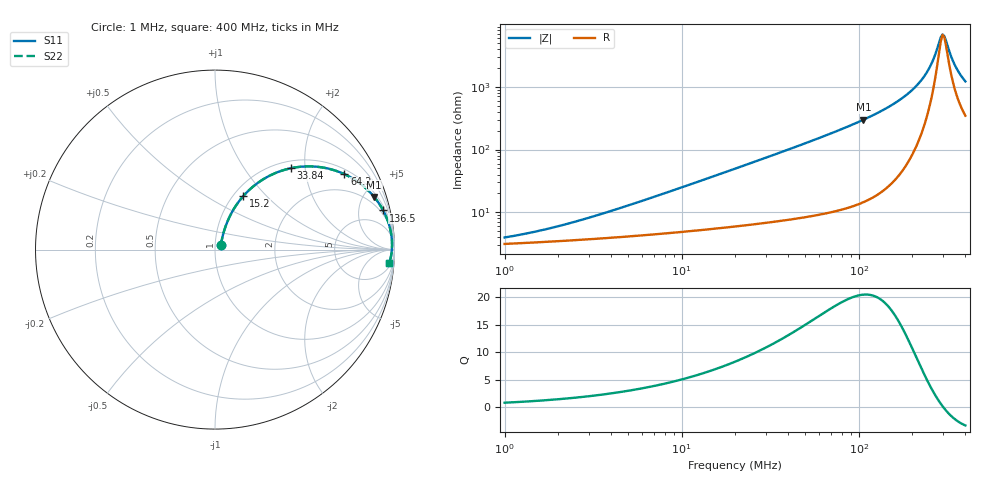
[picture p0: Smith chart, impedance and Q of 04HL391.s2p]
! Coilcraft 0402HL-391 Chip Inductor
! 20 July 2012
# MHz S MA R 50
!Freq  MagS11  AngS11  MagS21  AngS21  MagS12  AngS12  MagS22  AngS22
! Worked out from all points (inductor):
!   263 points, 1 MHz to 400 MHz, reference 50 ohm
!   read as one part in series: L = 390 nH near 5.189 MHz
!   highest Q = 20.5 at 106.2 MHz (marker M1), where L = 446 nH
!   self-resonance near 297.1 MHz
!   S11 on the Smith chart (normalised r, x): 1 MHz: 1.06, +0.05; 15.2 MHz: 1.11, +0.75; 33.84 MHz: 1.14, +1.68; 64.2 MHz: 1.19, +3.30; 136.5 MHz: 1.44, +8.45; 400 MHz: 8, -23
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1  0.03868 36.5  0.9692 -1.4  0.9692 -1.4  0.03868 36.5
1.616449  0.05026 47.4  0.9667 -2.2  0.9667 -2.2  0.05026 47.4
2.735188  0.07357 57.6  0.9626 -3.7  0.9626 -3.7  0.07357 57.6
7.481253  0.178 66.1  0.9422 -10.0  0.9422 -10.0  0.178 66.1
15.20028  0.3373 62.1  0.8936 -19.5  0.8936 -19.5  0.3373 62.1
20  0.4244 58.2  0.8559 -24.9  0.8559 -24.9  0.4244 58.2
33.84193  0.6192 47.0  0.7345 -38.1  0.7345 -38.1  0.6192 47.0
54.70376  0.7885 34.5  0.5674 -51.9  0.5674 -51.9  0.7885 34.5
64.20042  0.8344 30.3  0.5051 -56.4  0.5051 -56.4  0.8344 30.3
106.1772  0.9344 18.2  0.3135 -69.0  0.3135 -69.0  0.9344 18.2
136.5458  0.9622 13.1  0.2274 -73.9  0.2274 -73.9  0.9622 13.1
149.6251  0.9693 11.4  0.198 -75.4  0.198 -75.4  0.9693 11.4
192.4204  0.9824 7.0  0.1222 -78.2  0.1222 -78.2  0.9824 7.0
231.0486  0.9865 4.0  0.07094 -77.0  0.07094 -77.0  0.9865 4.0
259.0365  0.9871 2.2  0.0407 -70.3  0.0407 -70.3  0.9871 2.2
271.159  0.9868 1.5  0.02944 -62.7  0.02944 -62.7  0.9868 1.5
290.4147  0.986 0.5  0.01614 -29.8  0.01614 -29.8  0.986 0.5
297.1325  0.9856 0.1  0.01451 -8.0  0.01451 -8.0  0.9856 0.1
304.0057  0.9852 -0.2  0.01536 15.0  0.01536 15.0  0.9852 -0.2
333.1254  0.9827 -1.6  0.03299 57.5  0.03299 57.5  0.9827 -1.6
348.7152  0.981 -2.3  0.04432 63.5  0.04432 63.5  0.981 -2.3
400  0.9743 -4.4  0.08009 69.1  0.08009 69.1  0.9743 -4.4
